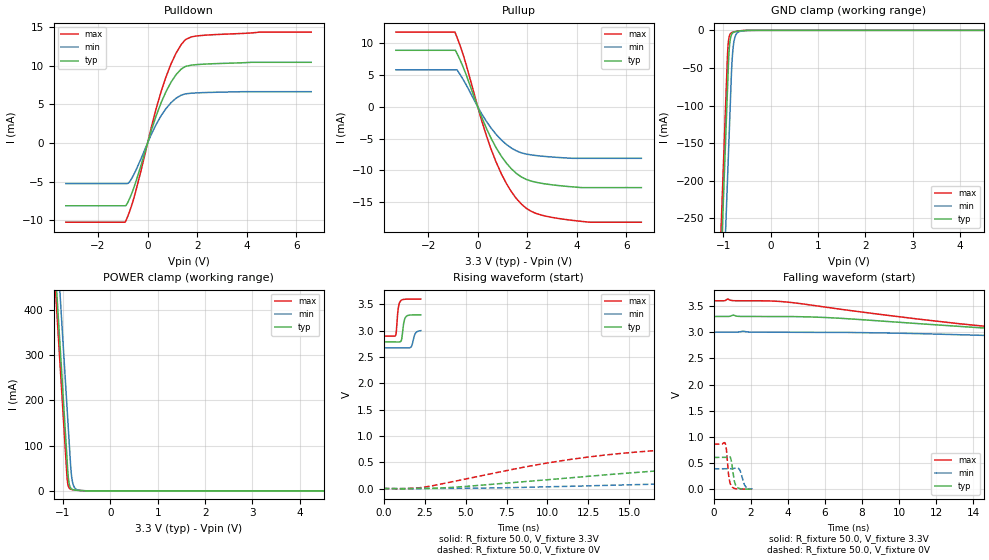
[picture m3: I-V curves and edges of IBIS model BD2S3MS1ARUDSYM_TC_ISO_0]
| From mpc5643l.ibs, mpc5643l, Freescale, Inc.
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| *** New cell (Generated with 5.14beta1 (Sep 20 2010 13:23:23))
[Model]   BD2S3MS1ARUDSYM_TC_ISO_0
Model_type I/O
Polarity   Non-Inverting
Enable   Active-Low
| CAP_THRESHOLD on pad pad is "CMOS" :
| Rising=10.0% of VDDE1   Falling=90.0% of VDDE1
| C_comp min and max val. don't necessarily correlate with the min and max pvt
| but are the smallest and greatest pad capacitance found.
| var   typ   min   max
C_comp   1.60298pF  1.53059pF  1.68637pF
Vinl = 1.05V | Dummy value overriden by next lines
Vinh = 2.34V | Dummy value overriden by next lines
Vmeas = 1.65V   | Reference voltage for timing measurements
Cref  = 25.0pF   | Timing specification test load capacitance value
Rref  = 1.0MOhm   | Timing specification test load resistance value
Vref  = 1.65V   | Timing specification test load voltage
[Model Spec]
| TIME_THRESHOLD on pin ipp_ind is "CORE" :
| Rising=40.0% of VDD   Falling=60.0% of VDD
Vinl 1.30950V 1.19650V 1.40650V
Vinh 1.89650V 1.72150V 2.04550V
| variable   typ   min   max
[Temperature Range] 25.0 150.0 -40.0
| variable   typ   min   max
[Voltage Range] 3.3V 3.0V 3.6V
| variable   typ   min   max
[POWER Clamp Reference] 3.3V 3.0V 3.6V
| variable   typ   min   max
[GND Clamp Reference] 0V 0V 0V
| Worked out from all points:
|   slope of the pulldown table from 0 to 0.495 V, typ, clamps not added: 103 ohm
|   slope of the pullup table from 0 to 0.495 V, typ, clamps not added: 108 ohm
|   GND clamp passes 1 mA (typ) near -0.68 V on its own axis
|   POWER clamp passes 1 mA (typ) near -0.66 V on its own axis
|   rising waveform, R_fixture 50.0, V_fixture 3.3V: 20-80 % time 136ps typ, 167ps min, 121ps max; typ from 2.79 V to 3.3 V
|   falling waveform, R_fixture 50.0, V_fixture 3.3V: 20-80 % time 15ns typ, 23.4ns min, 10.7ns max; typ from 3.3 V to 2.79 V
|   rising waveform, R_fixture 50.0, V_fixture 0V: 20-80 % time 17.6ns typ, 35.4ns min, 10.4ns max; typ from 0 V to 0.606 V
|   falling waveform, R_fixture 50.0, V_fixture 0V: 20-80 % time 161ps typ, 201ps min, 143ps max; typ from 0.606 V to 0 V
[POWER Clamp]
-3.3V     4.125A     4.239A     4.084A
-1.21V    572.2mA    686.2mA    530.8mA
-1.14V    453.2mA    567.2mA    411.8mA
-1.07V    334.2mA    448.2mA    292.8mA
-1V       215.2mA    329.2mA    173.8mA
-910mV    62.21mA    176.2mA    24.61mA
-880mV    22.38mA    125.2mA    8.495mA
-840mV    6.765mA    57.19mA    3.971mA
-810mV    3.645mA    26.2mA     3.059mA
-770mV    2.237mA    9.849mA    2.403mA
-610mV    694.5uA    892.2uA    750.7uA
6.6V      0A         0A         0A
[GND Clamp]
-3.3V     -4.141A    -4.261A    -4.095A
-1.08V    -366.6mA   -487mA     -321.3mA
-910mV    -77.61mA   -198mA     -32.34mA
-890mV    -43.61mA   -164mA     -14.22mA
-870mV    -21.62mA   -130mA     -7.309mA
-850mV    -11.35mA   -95.98mA   -4.558mA
-830mV    -6.494mA   -61.98mA   -3.352mA
-810mV    -4.133mA   -36.82mA   -2.724mA
-780mV    -2.546mA   -17.3mA    -2.152mA
-740mV    -1.678mA   -6.849mA   -1.597mA
-540mV    -211.7uA   -469.1uA   -127.2uA
6.6V      5.511nA    1.73uA     35.76pA
| variable   typ   min   max
[Pullup Reference] 3.3V 3.0V 3.6V
| variable   typ   min   max
[Pulldown Reference] 0V 0V 0V
[Pullup]
-3.3V     8.894mA    5.825mA    11.76mA
-920mV    8.894mA    5.825mA    11.76mA
-840mV    8.427mA    5.825mA    10.98mA
-530mV    5.674mA    3.9mA      7.457mA
340mV     -3.307mA   -2.24mA    -4.444mA
740mV     -6.433mA   -4.335mA   -8.693mA
950mV     -7.762mA   -5.212mA   -10.53mA
1.35V     -9.735mA   -6.478mA   -13.33mA
1.96V     -11.44mA   -7.45mA    -15.98mA
2.57V     -12.04mA   -7.766mA   -17.05mA
3.78V     -12.59mA   -8.103mA   -17.86mA
6.6V      -12.72mA   -8.114mA   -18.17mA
[Pulldown]
-3.3V     -8.133mA   -5.257mA   -10.26mA
-910mV    -8.133mA   -5.257mA   -10.26mA
-760mV    -7.434mA   -5.146mA   -9.165mA
-550mV    -5.747mA   -4.049mA   -7.092mA
340mV     3.466mA    2.369mA    4.386mA
740mV     6.626mA    4.438mA    8.531mA
1.15V     8.847mA    5.792mA    11.63mA
1.54V     9.906mA    6.354mA    13.39mA
1.76V     10.07mA    6.435mA    13.72mA
2.57V     10.24mA    6.543mA    13.99mA
4.52V     10.44mA    6.634mA    14.35mA
6.6V      10.44mA    6.634mA    14.35mA
[Ramp]
dV/dt_r 363.71646mV/17.63188ns 233.35792mV/35.39041ns 516.36339mV/10.37863ns
dV/dt_f 308.06866mV/14.96325ns 196.50546mV/23.39619ns 421.49291mV/10.6896ns
R_load = 50.0
| Removed startup time: 0s 0s 0s  .
| Removed end time: 2.267ns.
[Rising Waveform]
R_fixture   = 50.0
V_fixture   = 3.3V
V_fixture_min = 3.0V
V_fixture_max = 3.6V
0s        2.787V     2.672V     2.898V
729ps     2.787V     2.672V     2.911V
773ps     2.787V     2.672V     2.985V
888ps     2.785V     2.672V     3.419V
1.046ns   2.796V     2.672V     3.569V
1.236ns   3.164V     2.672V     3.594V
1.356ns   3.262V     2.672V     3.597V
1.674ns   3.297V     2.691V     3.599V
1.93ns    3.299V     2.945V     3.599V
2.269ns   3.3V       3V         3.6V
| Removed startup time: 0s 0s 0s  .
| Removed end time: 103.9ns.
[Falling Waveform]
R_fixture   = 50.0
V_fixture   = 3.3V
V_fixture_min = 3.0V
V_fixture_max = 3.6V
0s        3.3V       3V         3.6V
750ps     3.299V     3V         3.633V
1.05ns    3.325V     2.999V     3.602V
4ns       3.3V       3V         3.574V
10.8ns    3.169V     2.974V     3.26V
16.65ns   3.033V     2.918V     3.05V
23.45ns   2.905V     2.851V     2.947V
31.4ns    2.836V     2.78V      2.918V
45.4ns    2.803V     2.715V     2.903V
104ns     2.787V     2.672V     2.898V
| Removed startup time: 0s 0s 0s  .
| Removed end time: 123.35ns.
[Rising Waveform]
R_fixture   = 50.0
V_fixture   = 0V
V_fixture_min = 0V
V_fixture_max = 0V
0s        15.53nV    1.006uV    13.79nV
850ps     501.9uV    980.8nV    -11.91mV
2.5ns     1.79mV     122.9uV    27.27mV
9.5ns     153.8mV    28.84mV    459.3mV
13.65ns   263mV      59.77mV    640.6mV
18.25ns   367.6mV    97.2mV     753.6mV
24.25ns   465.3mV    147.8mV    818.8mV
38.6ns    568.9mV    251.3mV    855.4mV
60.95ns   600.9mV    339.6mV    860.1mV
123.5ns   606.2mV    388.9mV    860.6mV
| Removed startup time: 0s 0s 0s  .
| Removed end time: 2.069ns.
[Falling Waveform]
R_fixture   = 50.0
V_fixture   = 0V
V_fixture_min = 0V
V_fixture_max = 0V
0s        606.2mV    389.2mV    860.6mV
619ps     606.3mV    389.2mV    872.8mV
681ps     611.3mV    389.1mV    761.1mV
820ps     631.9mV    388.9mV    220.7mV
979ps     471.6mV    389.7mV    46.07mV
1.102ns   166.6mV    397.3mV    15.24mV
1.234ns   47.85mV    408.1mV    5.03mV
1.417ns   10.1mV     357.1mV    1.41mV
1.704ns   1.391mV    55.72mV    353.9uV
2.071ns   96.99uV    51.44uV    122.1uV
